(* Logix 5000 AddOnInstructionDefinition export Banner_EZAK2_Param_v4; software revision 33.00; part 2 of 3 *)
(* tags used below, declared in another part *)
   EZAK2 : Banner_EZAK2_v4;
   Port_Data : Banner_IOL_Port_v4;
   Port : DINT;
   Local_Control : DINT;
   Command_Being_Processed : BOOL;
   Update_Archive : BOOL;
   Index_Write_Control : DINT;
   Index_Write_Inprocess : INT;
   Inprocess_Index : DINT;
(* Banner_EZAK2_Param_v4, continued *)

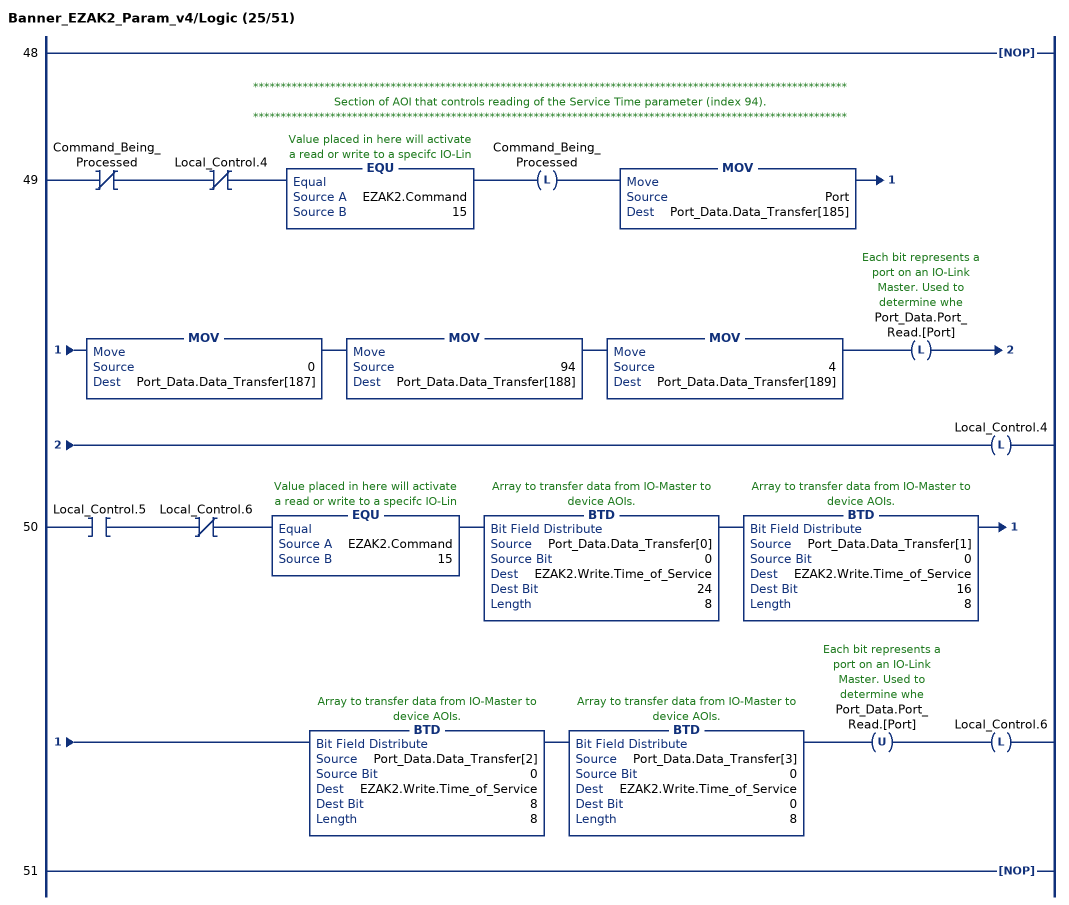
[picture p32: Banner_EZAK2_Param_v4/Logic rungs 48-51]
   48: NOP();
   // ************************************************************************************************************
   // Section of AOI that controls reading of the Service Time parameter (index 94).
   // ************************************************************************************************************
   49: XIO(Command_Being_Processed)XIO(Local_Control.4)EQU(EZAK2.Command,15)OTL(Command_Being_Processed)MOV(Port,Port_Data.Data_Transfer[185])MOV(0,Port_Data.Data_Transfer[187])MOV(94,Port_Data.Data_Transfer[188])MOV(4,Port_Data.Data_Transfer[189])OTL(Port_Data.Port_Read.[Port])OTL(Local_Control.4);
   50: XIC(Local_Control.5)XIO(Local_Control.6)EQU(EZAK2.Command,15)BTD(Port_Data.Data_Transfer[0],0,EZAK2.Write.Time_of_Service,24,8)BTD(Port_Data.Data_Transfer[1],0,EZAK2.Write.Time_of_Service,16,8)BTD(Port_Data.Data_Transfer[2],0,EZAK2.Write.Time_of_Service,8,8)BTD(Port_Data.Data_Transfer[3],0,EZAK2.Write.Time_of_Service,0,8)OTU(Port_Data.Port_Read.[Port])OTL(Local_Control.6);
   51: NOP();
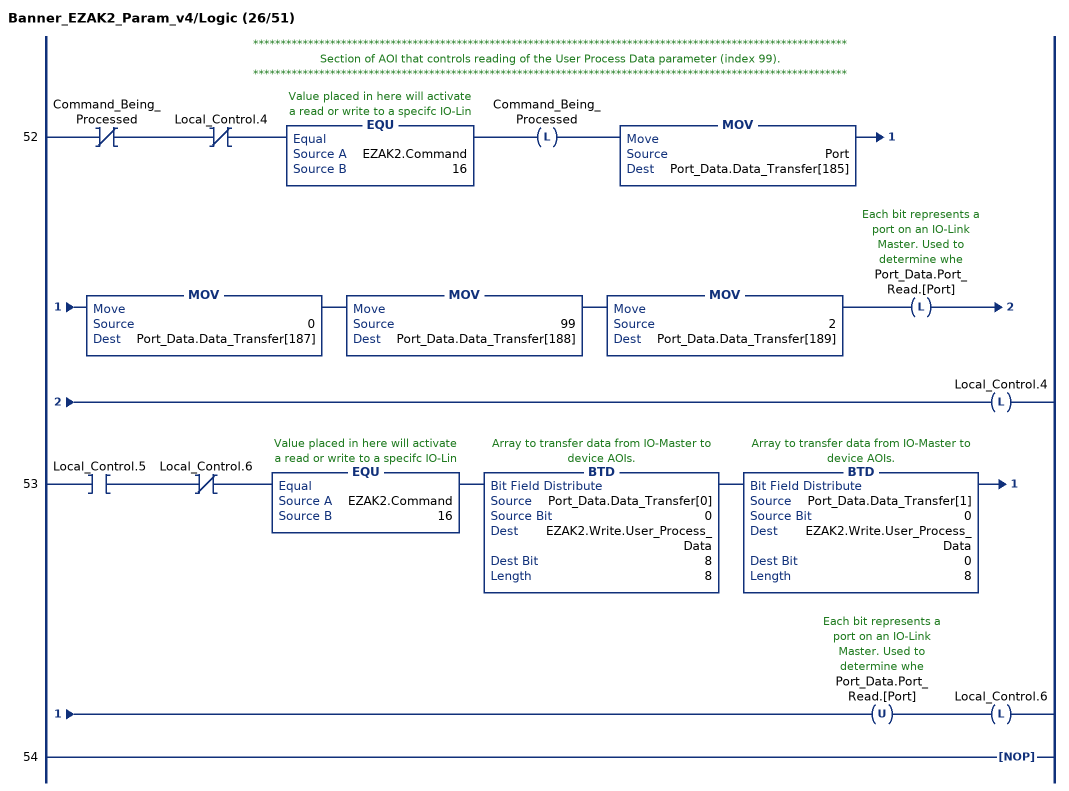
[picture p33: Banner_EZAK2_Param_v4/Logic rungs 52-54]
   // ************************************************************************************************************
   // Section of AOI that controls reading of the User Process Data parameter (index 99).
   // ************************************************************************************************************
   52: XIO(Command_Being_Processed)XIO(Local_Control.4)EQU(EZAK2.Command,16)OTL(Command_Being_Processed)MOV(Port,Port_Data.Data_Transfer[185])MOV(0,Port_Data.Data_Transfer[187])MOV(99,Port_Data.Data_Transfer[188])MOV(2,Port_Data.Data_Transfer[189])OTL(Port_Data.Port_Read.[Port])OTL(Local_Control.4);
   53: XIC(Local_Control.5)XIO(Local_Control.6)EQU(EZAK2.Command,16)BTD(Port_Data.Data_Transfer[0],0,EZAK2.Write.User_Process_Data,8,8)BTD(Port_Data.Data_Transfer[1],0,EZAK2.Write.User_Process_Data,0,8)OTU(Port_Data.Port_Read.[Port])OTL(Local_Control.6);
   54: NOP();
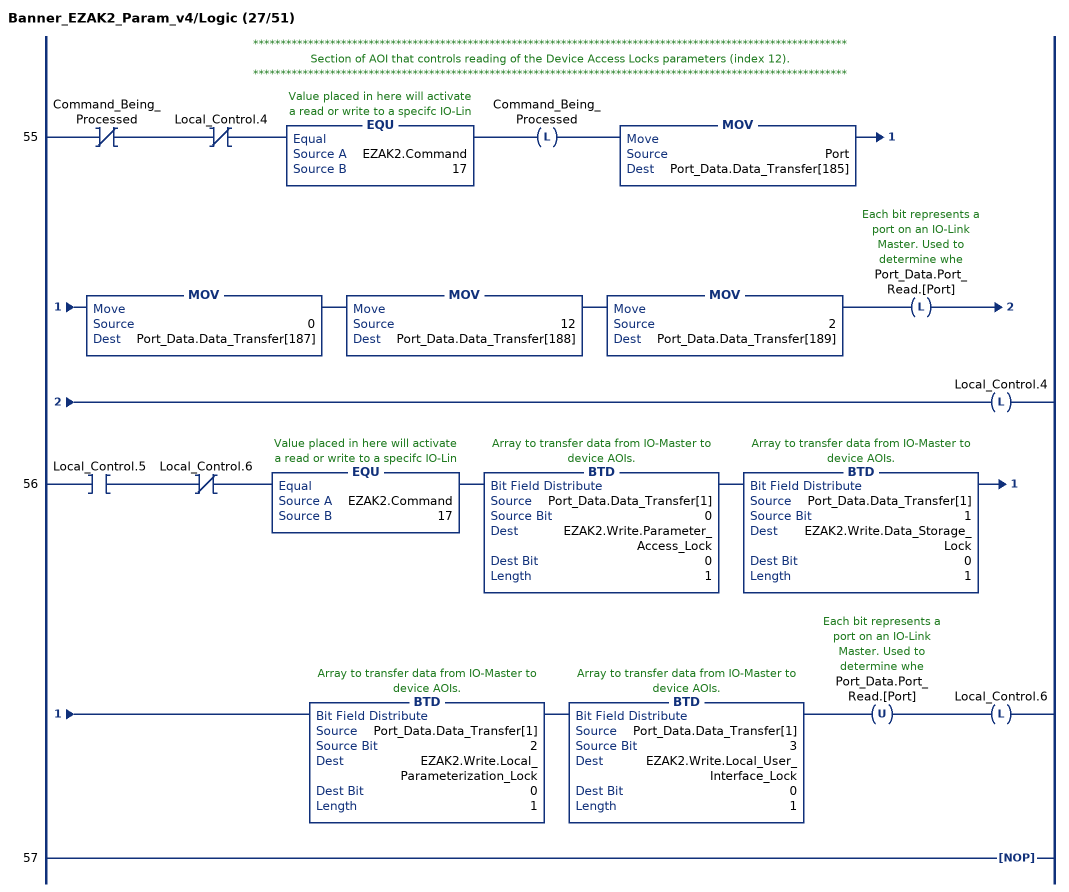
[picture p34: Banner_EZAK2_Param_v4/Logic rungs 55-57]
   // ************************************************************************************************************
   // Section of AOI that controls reading of the Device Access Locks parameters (index 12).
   // ************************************************************************************************************
   55: XIO(Command_Being_Processed)XIO(Local_Control.4)EQU(EZAK2.Command,17)OTL(Command_Being_Processed)MOV(Port,Port_Data.Data_Transfer[185])MOV(0,Port_Data.Data_Transfer[187])MOV(12,Port_Data.Data_Transfer[188])MOV(2,Port_Data.Data_Transfer[189])OTL(Port_Data.Port_Read.[Port])OTL(Local_Control.4);
   56: XIC(Local_Control.5)XIO(Local_Control.6)EQU(EZAK2.Command,17)BTD(Port_Data.Data_Transfer[1],0,EZAK2.Write.Parameter_Access_Lock,0,1)BTD(Port_Data.Data_Transfer[1],1,EZAK2.Write.Data_Storage_Lock,0,1)BTD(Port_Data.Data_Transfer[1],2,EZAK2.Write.Local_Parameterization_Lock,0,1)BTD(Port_Data.Data_Transfer[1],3,EZAK2.Write.Local_User_Interface_Lock,0,1)OTU(Port_Data.Port_Read.[Port])OTL(Local_Control.6);
   57: NOP();
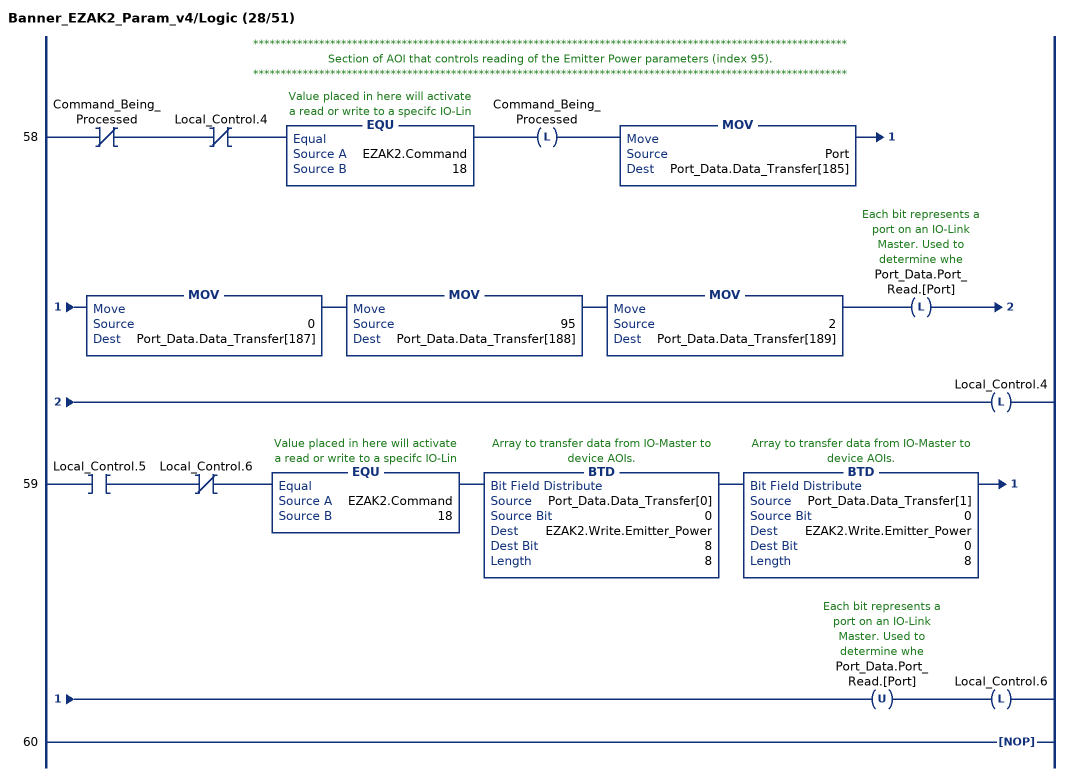
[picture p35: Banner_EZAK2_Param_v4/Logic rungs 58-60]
   // ************************************************************************************************************
   // Section of AOI that controls reading of the Emitter Power parameters (index 95).
   // ************************************************************************************************************
   58: XIO(Command_Being_Processed)XIO(Local_Control.4)EQU(EZAK2.Command,18)OTL(Command_Being_Processed)MOV(Port,Port_Data.Data_Transfer[185])MOV(0,Port_Data.Data_Transfer[187])MOV(95,Port_Data.Data_Transfer[188])MOV(2,Port_Data.Data_Transfer[189])OTL(Port_Data.Port_Read.[Port])OTL(Local_Control.4);
   59: XIC(Local_Control.5)XIO(Local_Control.6)EQU(EZAK2.Command,18)BTD(Port_Data.Data_Transfer[0],0,EZAK2.Write.Emitter_Power,8,8)BTD(Port_Data.Data_Transfer[1],0,EZAK2.Write.Emitter_Power,0,8)OTU(Port_Data.Port_Read.[Port])OTL(Local_Control.6);
   60: NOP();
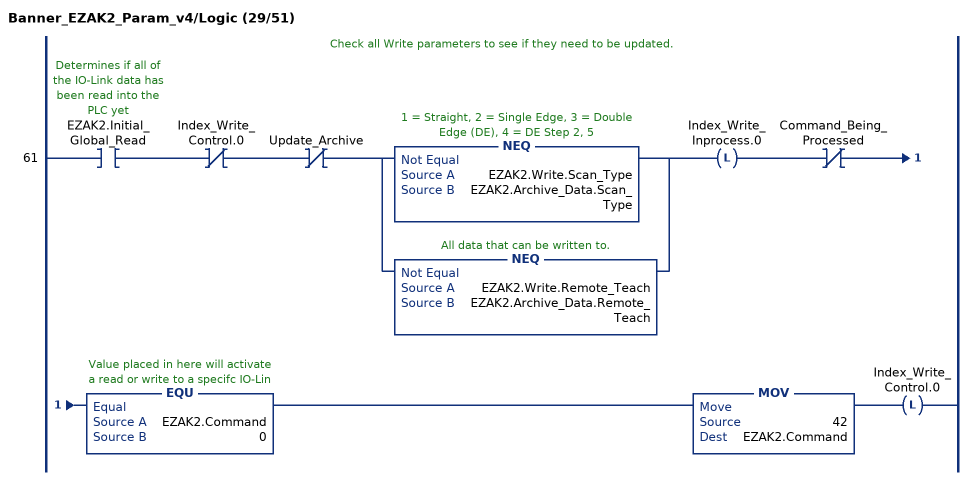
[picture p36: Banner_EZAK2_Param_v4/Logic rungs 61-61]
   // Check all Write parameters to see if they need to be updated.
   61: XIC(EZAK2.Initial_Global_Read)XIO(Index_Write_Control.0)XIO(Update_Archive)[NEQ(EZAK2.Write.Scan_Type,EZAK2.Archive_Data.Scan_Type) ,NEQ(EZAK2.Write.Remote_Teach,EZAK2.Archive_Data.Remote_Teach) ]OTL(Index_Write_Inprocess.0)XIO(Command_Being_Processed)EQU(EZAK2.Command,0)MOV(42,EZAK2.Command)OTL(Index_Write_Control.0);
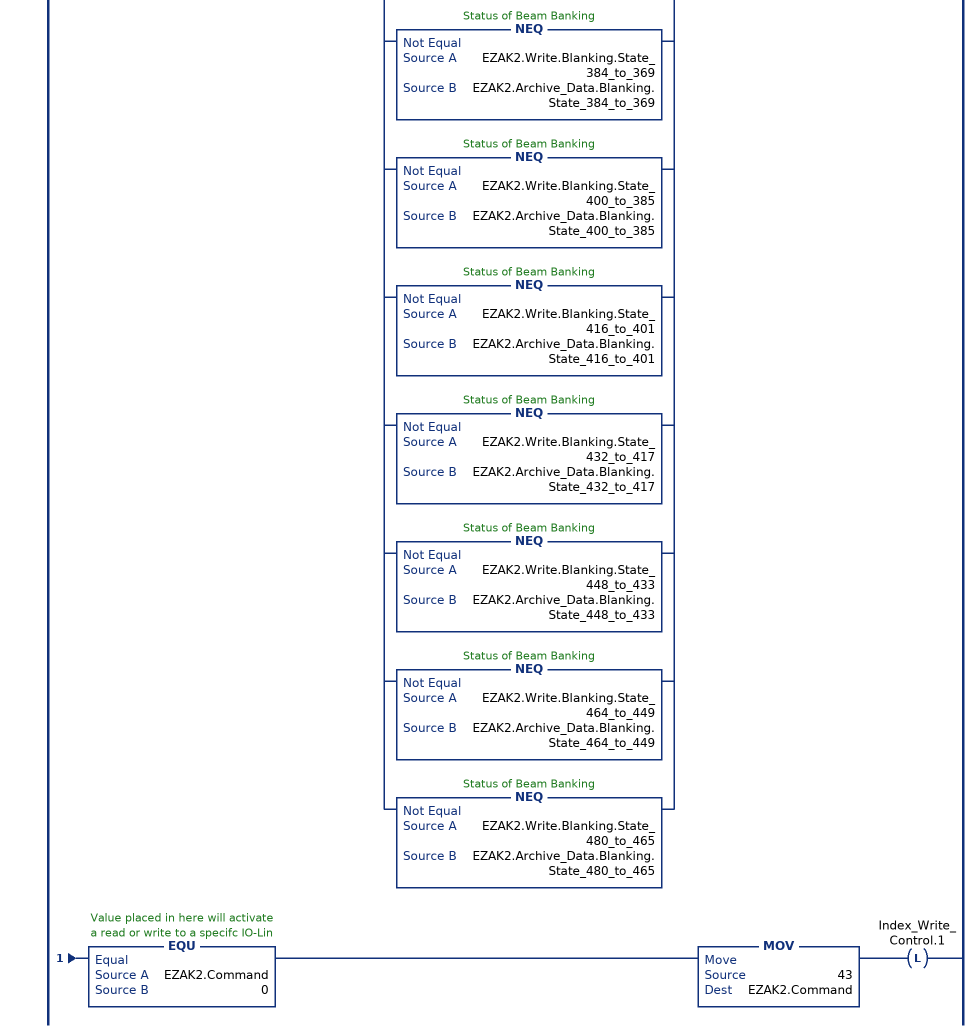
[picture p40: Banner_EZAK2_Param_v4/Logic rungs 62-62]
   62: XIC(EZAK2.Initial_Global_Read)XIO(Index_Write_Control.1)XIO(Update_Archive)[NEQ(EZAK2.Write.Blanking.State_16_to_1,EZAK2.Archive_Data.Blanking.State_16_to_1) ,NEQ(EZAK2.Write.Blanking.State_32_to_17,EZAK2.Archive_Data.Blanking.State_32_to_17) ,NEQ(EZAK2.Write.Blanking.State_48_to_33,EZAK2.Archive_Data.Blanking.State_48_to_33) ,NEQ(EZAK2.Write.Blanking.State_64_to_49,EZAK2.Archive_Data.Blanking.State_64_to_49) ,NEQ(EZAK2.Write.Blanking.State_80_to_65,EZAK2.Archive_Data.Blanking.State_80_to_65) ,NEQ(EZAK2.Write.Blanking.State_96_to_81,EZAK2.Archive_Data.Blanking.State_96_to_81) ,NEQ(EZAK2.Write.Blanking.State_112_to_97,EZAK2.Archive_Data.Blanking.State_112_to_97) ,NEQ(EZAK2.Write.Blanking.State_128_to_113,EZAK2.Archive_Data.Blanking.State_128_to_113) ,NEQ(EZAK2.Write.Blanking.State_144_to_129,EZAK2.Archive_Data.Blanking.State_144_to_129) ,NEQ(EZAK2.Write.Blanking.State_160_to_145,EZAK2.Archive_Data.Blanking.State_160_to_145) ,NEQ(EZAK2.Write.Blanking.State_176_to_161,EZAK2.Archive_Data.Blanking.State_176_to_161) ,NEQ(EZAK2.Write.Blanking.State_192_to_177,EZAK2.Archive_Data.Blanking.State_192_to_177) ,NEQ(EZAK2.Write.Blanking.State_208_to_193,EZAK2.Archive_Data.Blanking.State_208_to_193) ,NEQ(EZAK2.Write.Blanking.State_224_to_209,EZAK2.Archive_Data.Blanking.State_224_to_209) ,NEQ(EZAK2.Write.Blanking.State_240_to_225,EZAK2.Archive_Data.Blanking.State_240_to_225) ,NEQ(EZAK2.Write.Blanking.State_256_to_241,EZAK2.Archive_Data.Blanking.State_256_to_241) ,NEQ(EZAK2.Write.Blanking.State_272_to_257,EZAK2.Archive_Data.Blanking.State_272_to_257) ,NEQ(EZAK2.Write.Blanking.State_288_to_273,EZAK2.Archive_Data.Blanking.State_288_to_273) ,NEQ(EZAK2.Write.Blanking.State_304_to_289,EZAK2.Archive_Data.Blanking.State_304_to_289) ,NEQ(EZAK2.Write.Blanking.State_320_to_305,EZAK2.Archive_Data.Blanking.State_320_to_305) ,NEQ(EZAK2.Write.Blanking.State_336_to_321,EZAK2.Archive_Data.Blanking.State_336_to_321) ,NEQ(EZAK2.Write.Blanking.State_352_to_337,EZAK2.Archive_Data.Blanking.State_352_to_337) ,NEQ(EZAK2.Write.Blanking.State_368_to_353,EZAK2.Archive_Data.Blanking.State_368_to_353) ,NEQ(EZAK2.Write.Blanking.State_384_to_369,EZAK2.Archive_Data.Blanking.State_384_to_369) ,NEQ(EZAK2.Write.Blanking.State_400_to_385,EZAK2.Archive_Data.Blanking.State_400_to_385) ,NEQ(EZAK2.Write.Blanking.State_416_to_401,EZAK2.Archive_Data.Blanking.State_416_to_401) ,NEQ(EZAK2.Write.Blanking.State_432_to_417,EZAK2.Archive_Data.Blanking.State_432_to_417) ,NEQ(EZAK2.Write.Blanking.State_448_to_433,EZAK2.Archive_Data.Blanking.State_448_to_433) ,NEQ(EZAK2.Write.Blanking.State_464_to_449,EZAK2.Archive_Data.Blanking.State_464_to_449) ,NEQ(EZAK2.Write.Blanking.State_480_to_465,EZAK2.Archive_Data.Blanking.State_480_to_465) ]OTL(Index_Write_Inprocess.1)XIO(Command_Being_Processed)EQU(EZAK2.Command,0)MOV(43,EZAK2.Command)OTL(Index_Write_Control.1);
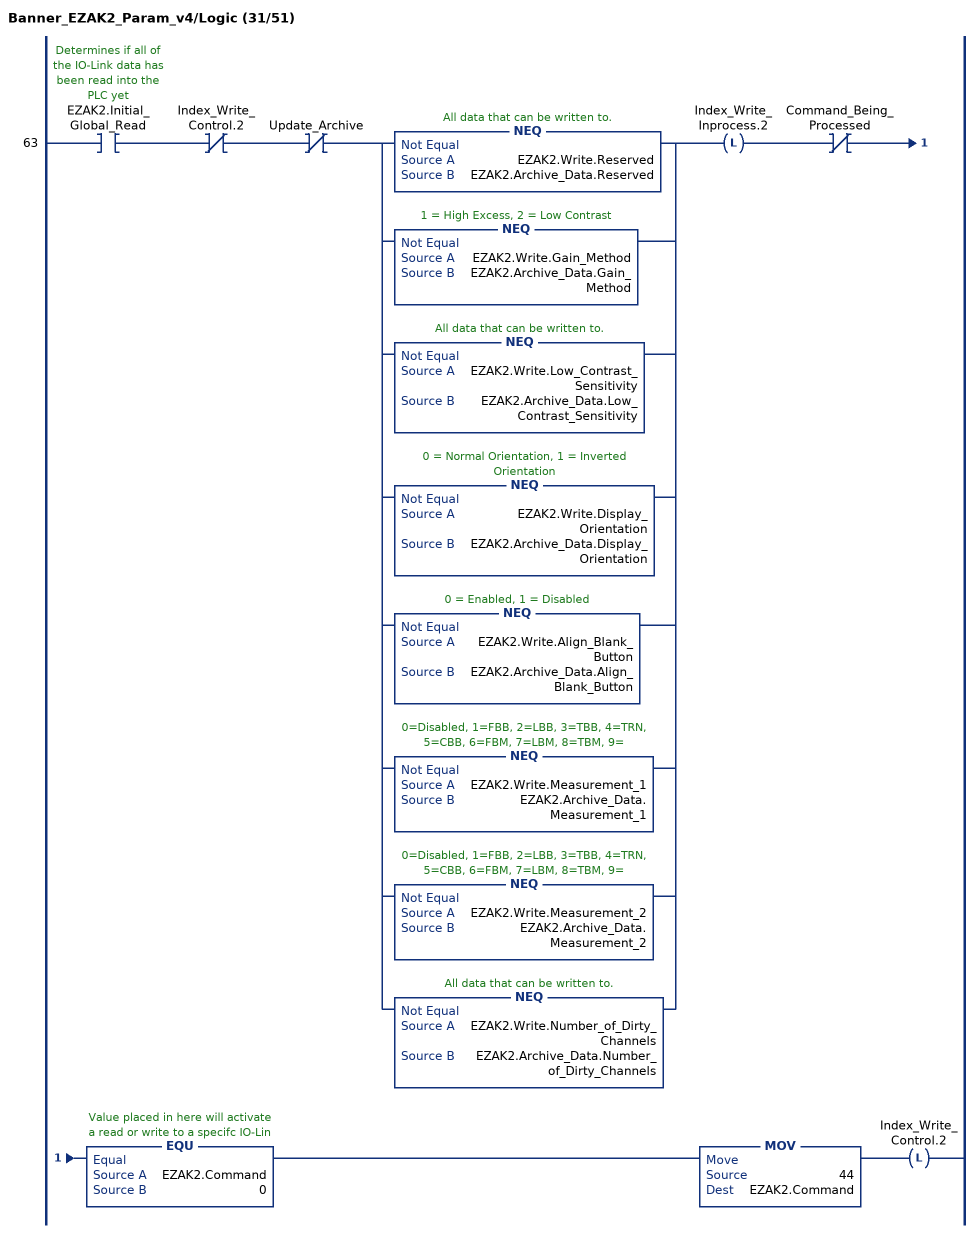
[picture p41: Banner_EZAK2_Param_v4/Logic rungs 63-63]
   63: XIC(EZAK2.Initial_Global_Read)XIO(Index_Write_Control.2)XIO(Update_Archive)[NEQ(EZAK2.Write.Reserved,EZAK2.Archive_Data.Reserved) ,NEQ(EZAK2.Write.Gain_Method,EZAK2.Archive_Data.Gain_Method) ,NEQ(EZAK2.Write.Low_Contrast_Sensitivity,EZAK2.Archive_Data.Low_Contrast_Sensitivity) ,NEQ(EZAK2.Write.Display_Orientation,EZAK2.Archive_Data.Display_Orientation) ,NEQ(EZAK2.Write.Align_Blank_Button,EZAK2.Archive_Data.Align_Blank_Button) ,NEQ(EZAK2.Write.Measurement_1,EZAK2.Archive_Data.Measurement_1) ,NEQ(EZAK2.Write.Measurement_2,EZAK2.Archive_Data.Measurement_2) ,NEQ(EZAK2.Write.Number_of_Dirty_Channels,EZAK2.Archive_Data.Number_of_Dirty_Channels) ]OTL(Index_Write_Inprocess.2)XIO(Command_Being_Processed)EQU(EZAK2.Command,0)MOV(44,EZAK2.Command)OTL(Index_Write_Control.2);
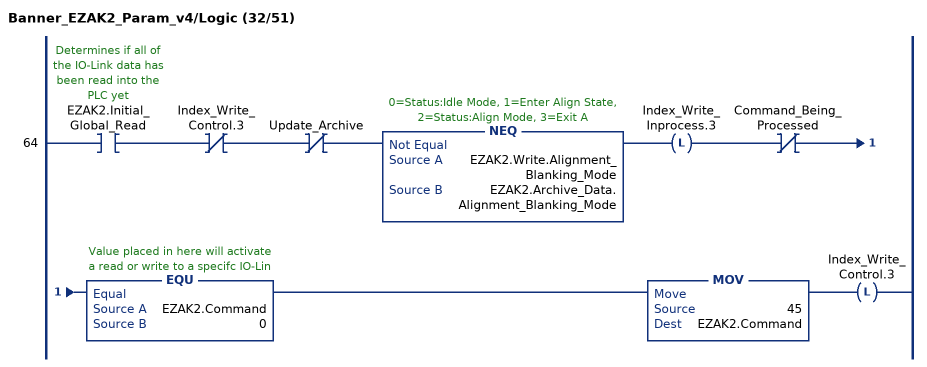
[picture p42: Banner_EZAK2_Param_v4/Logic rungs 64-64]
   64: XIC(EZAK2.Initial_Global_Read)XIO(Index_Write_Control.3)XIO(Update_Archive)NEQ(EZAK2.Write.Alignment_Blanking_Mode,EZAK2.Archive_Data.Alignment_Blanking_Mode)OTL(Index_Write_Inprocess.3)XIO(Command_Being_Processed)EQU(EZAK2.Command,0)MOV(45,EZAK2.Command)OTL(Index_Write_Control.3);
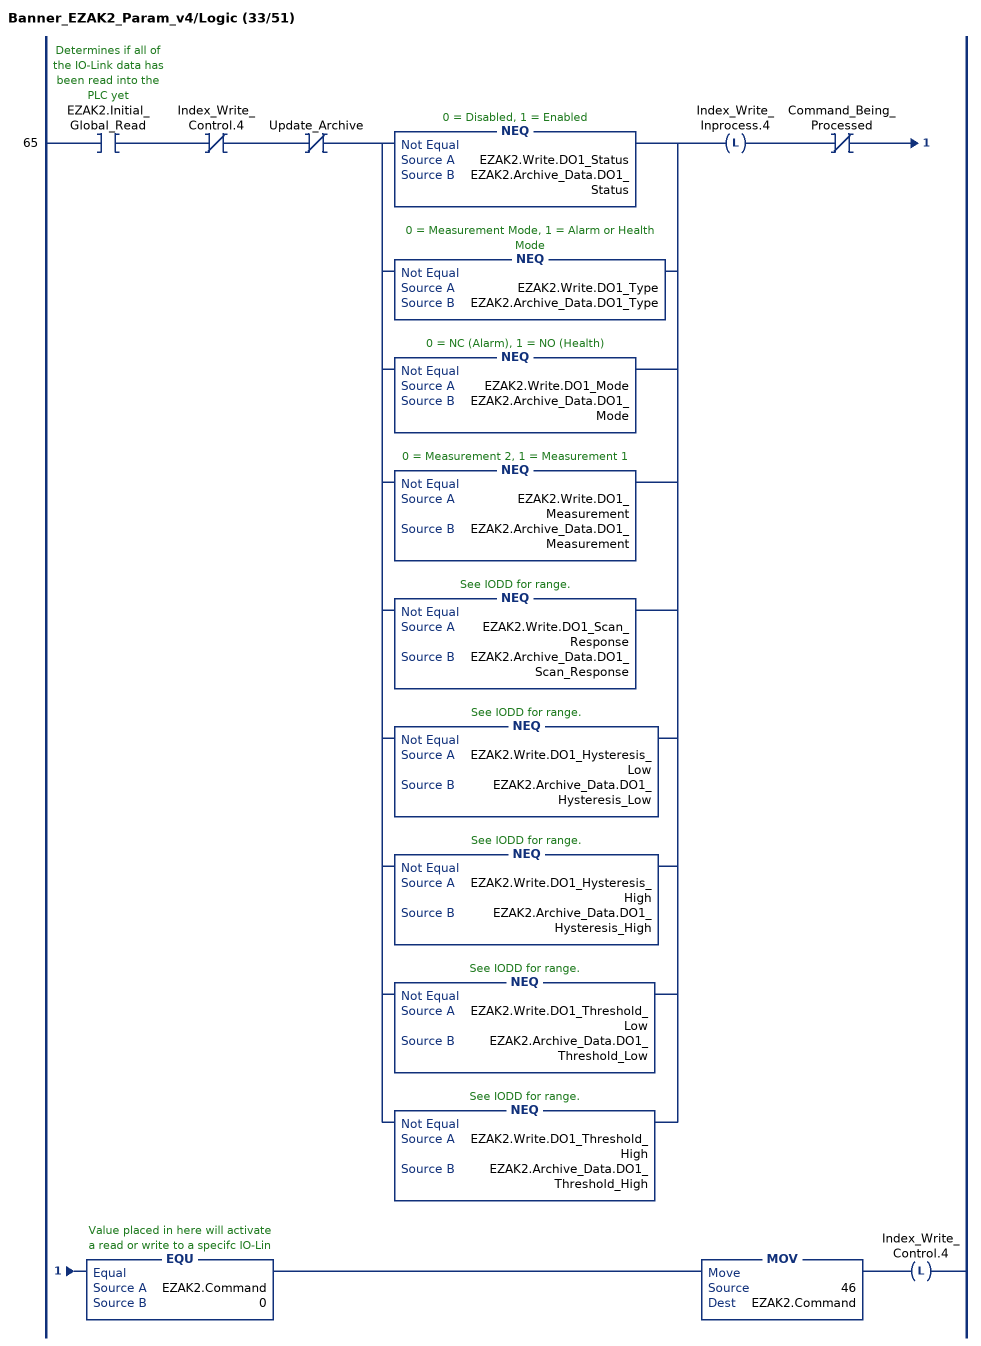
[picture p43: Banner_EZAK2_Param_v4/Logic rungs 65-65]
   65: XIC(EZAK2.Initial_Global_Read)XIO(Index_Write_Control.4)XIO(Update_Archive)[NEQ(EZAK2.Write.DO1_Status,EZAK2.Archive_Data.DO1_Status) ,NEQ(EZAK2.Write.DO1_Type,EZAK2.Archive_Data.DO1_Type) ,NEQ(EZAK2.Write.DO1_Mode,EZAK2.Archive_Data.DO1_Mode) ,NEQ(EZAK2.Write.DO1_Measurement,EZAK2.Archive_Data.DO1_Measurement) ,NEQ(EZAK2.Write.DO1_Scan_Response,EZAK2.Archive_Data.DO1_Scan_Response) ,NEQ(EZAK2.Write.DO1_Hysteresis_Low,EZAK2.Archive_Data.DO1_Hysteresis_Low) ,NEQ(EZAK2.Write.DO1_Hysteresis_High,EZAK2.Archive_Data.DO1_Hysteresis_High) ,NEQ(EZAK2.Write.DO1_Threshold_Low,EZAK2.Archive_Data.DO1_Threshold_Low) ,NEQ(EZAK2.Write.DO1_Threshold_High,EZAK2.Archive_Data.DO1_Threshold_High) ]OTL(Index_Write_Inprocess.4)XIO(Command_Being_Processed)EQU(EZAK2.Command,0)MOV(46,EZAK2.Command)OTL(Index_Write_Control.4);
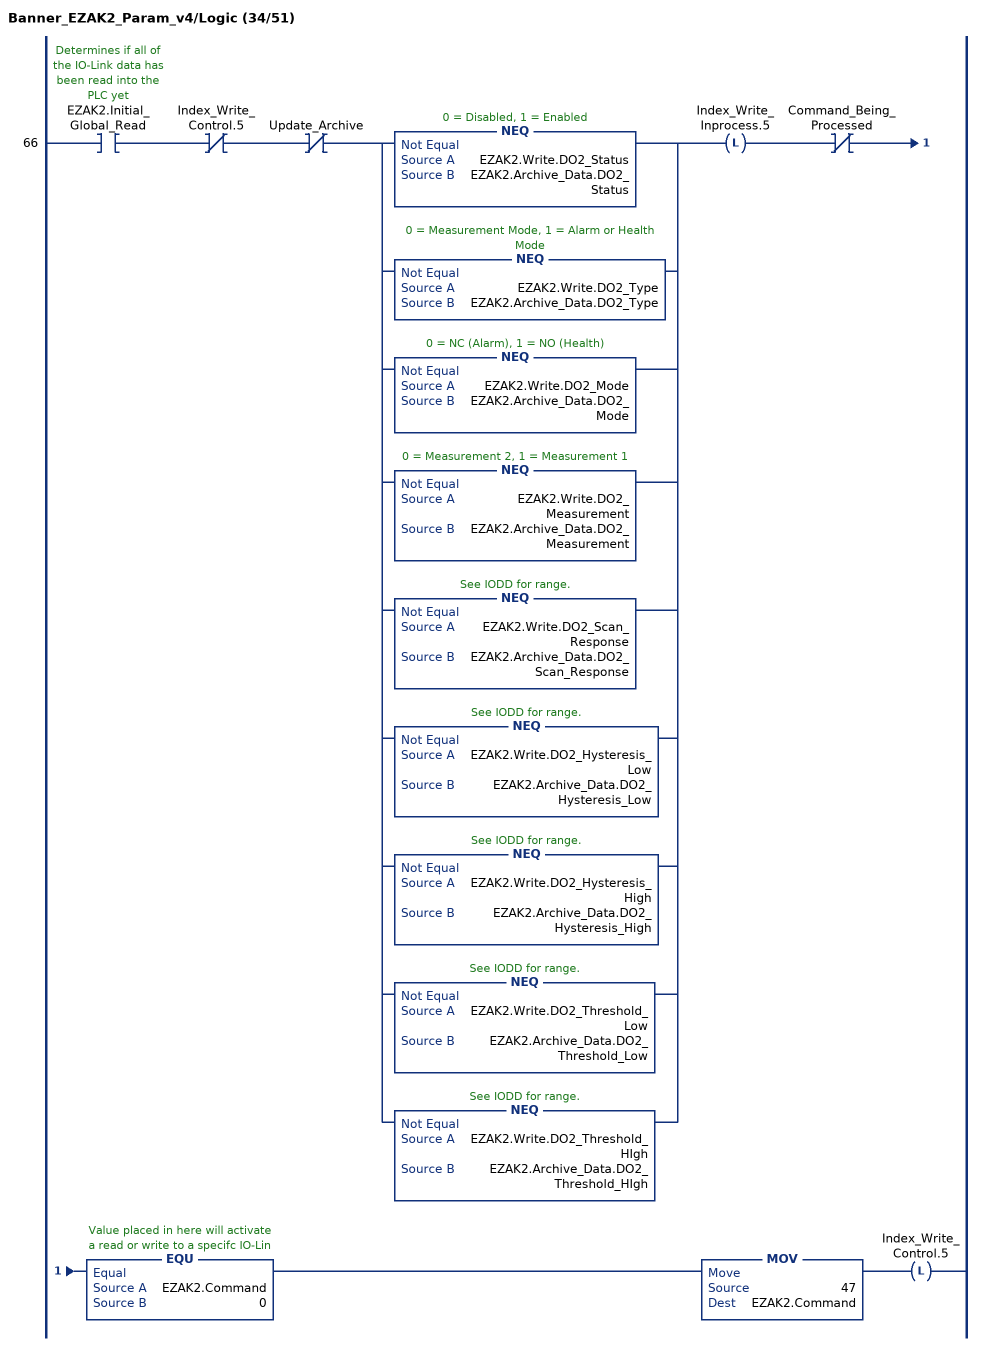
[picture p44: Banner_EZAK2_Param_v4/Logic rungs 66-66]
   66: XIC(EZAK2.Initial_Global_Read)XIO(Index_Write_Control.5)XIO(Update_Archive)[NEQ(EZAK2.Write.DO2_Status,EZAK2.Archive_Data.DO2_Status) ,NEQ(EZAK2.Write.DO2_Type,EZAK2.Archive_Data.DO2_Type) ,NEQ(EZAK2.Write.DO2_Mode,EZAK2.Archive_Data.DO2_Mode) ,NEQ(EZAK2.Write.DO2_Measurement,EZAK2.Archive_Data.DO2_Measurement) ,NEQ(EZAK2.Write.DO2_Scan_Response,EZAK2.Archive_Data.DO2_Scan_Response) ,NEQ(EZAK2.Write.DO2_Hysteresis_Low,EZAK2.Archive_Data.DO2_Hysteresis_Low) ,NEQ(EZAK2.Write.DO2_Hysteresis_High,EZAK2.Archive_Data.DO2_Hysteresis_High) ,NEQ(EZAK2.Write.DO2_Threshold_Low,EZAK2.Archive_Data.DO2_Threshold_Low) ,NEQ(EZAK2.Write.DO2_Threshold_HIgh,EZAK2.Archive_Data.DO2_Threshold_HIgh) ]OTL(Index_Write_Inprocess.5)XIO(Command_Being_Processed)EQU(EZAK2.Command,0)MOV(47,EZAK2.Command)OTL(Index_Write_Control.5);
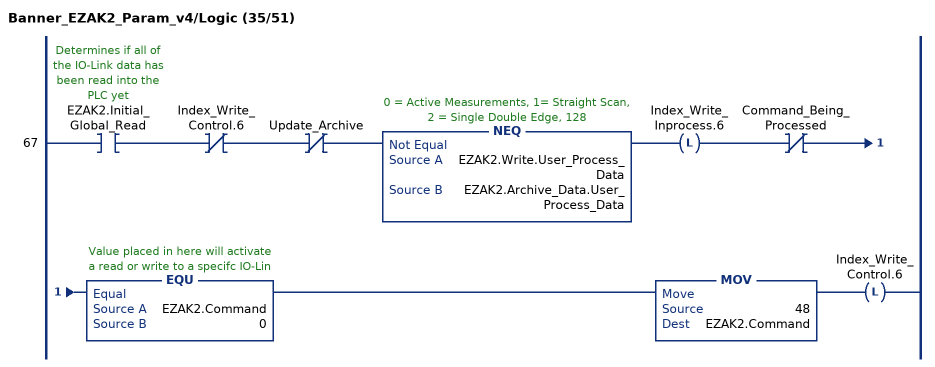
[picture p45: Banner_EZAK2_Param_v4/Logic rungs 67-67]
   67: XIC(EZAK2.Initial_Global_Read)XIO(Index_Write_Control.6)XIO(Update_Archive)NEQ(EZAK2.Write.User_Process_Data,EZAK2.Archive_Data.User_Process_Data)OTL(Index_Write_Inprocess.6)XIO(Command_Being_Processed)EQU(EZAK2.Command,0)MOV(48,EZAK2.Command)OTL(Index_Write_Control.6);
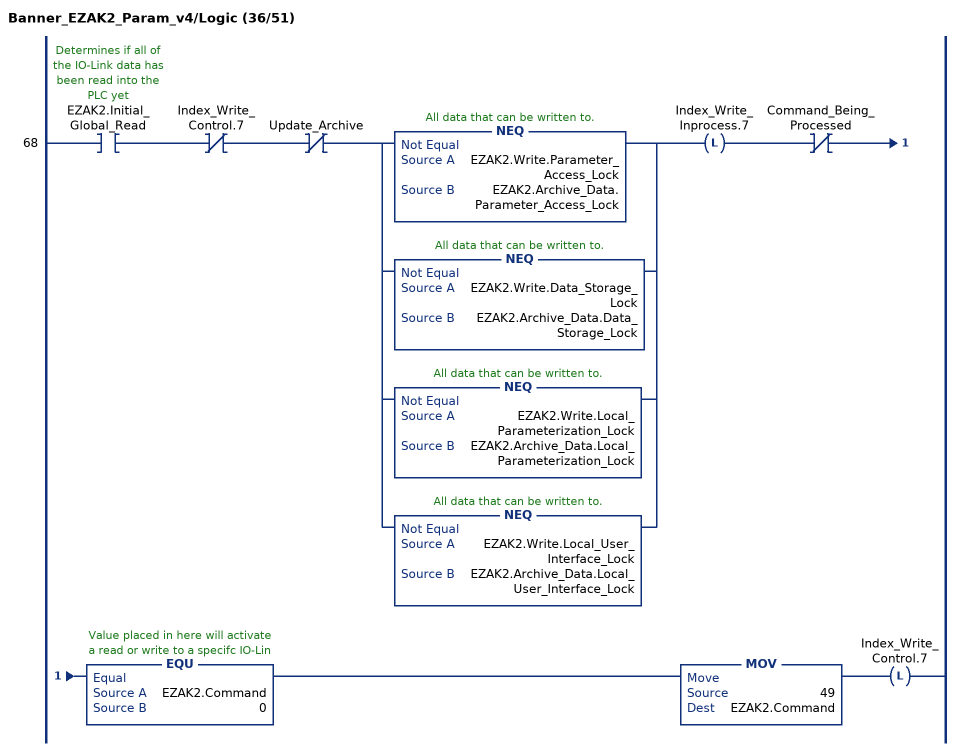
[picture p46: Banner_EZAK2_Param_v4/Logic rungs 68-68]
   68: XIC(EZAK2.Initial_Global_Read)XIO(Index_Write_Control.7)XIO(Update_Archive)[NEQ(EZAK2.Write.Parameter_Access_Lock,EZAK2.Archive_Data.Parameter_Access_Lock) ,NEQ(EZAK2.Write.Data_Storage_Lock,EZAK2.Archive_Data.Data_Storage_Lock) ,NEQ(EZAK2.Write.Local_Parameterization_Lock,EZAK2.Archive_Data.Local_Parameterization_Lock) ,NEQ(EZAK2.Write.Local_User_Interface_Lock,EZAK2.Archive_Data.Local_User_Interface_Lock) ]OTL(Index_Write_Inprocess.7)XIO(Command_Being_Processed)EQU(EZAK2.Command,0)MOV(49,EZAK2.Command)OTL(Index_Write_Control.7);
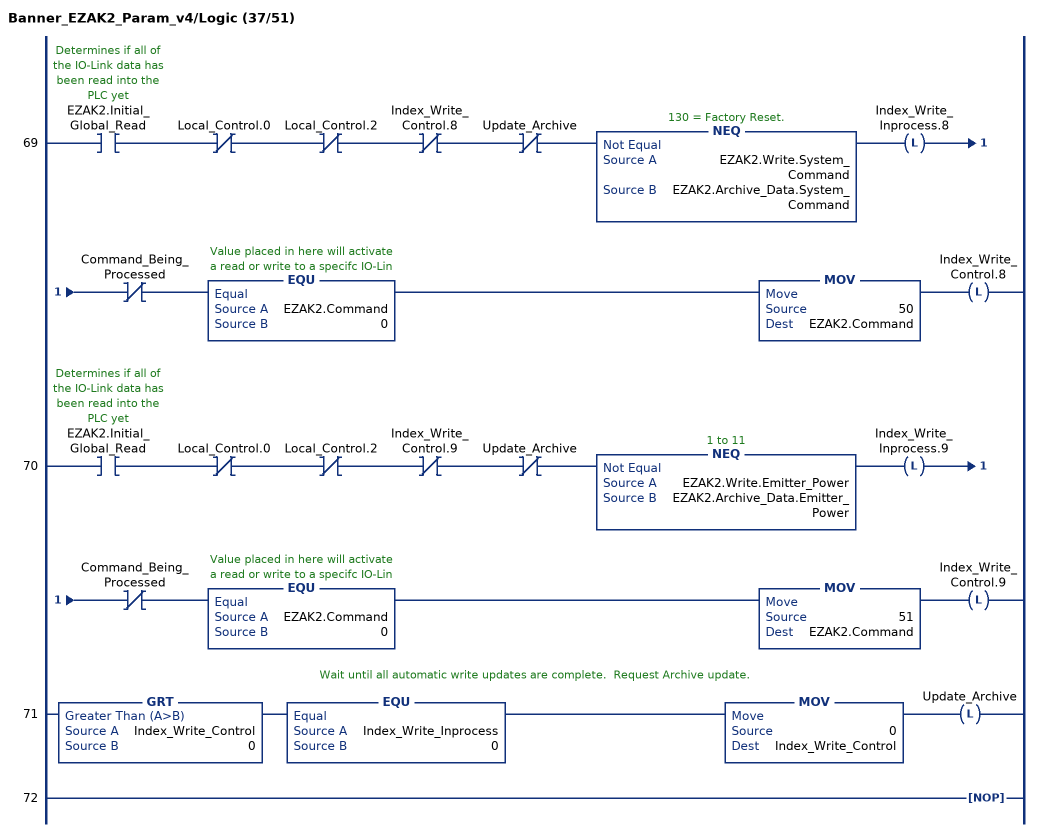
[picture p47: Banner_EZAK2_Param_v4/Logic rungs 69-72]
   69: XIC(EZAK2.Initial_Global_Read)XIO(Local_Control.0)XIO(Local_Control.2)XIO(Index_Write_Control.8)XIO(Update_Archive)NEQ(EZAK2.Write.System_Command,EZAK2.Archive_Data.System_Command)OTL(Index_Write_Inprocess.8)XIO(Command_Being_Processed)EQU(EZAK2.Command,0)MOV(50,EZAK2.Command)OTL(Index_Write_Control.8);
   70: XIC(EZAK2.Initial_Global_Read)XIO(Local_Control.0)XIO(Local_Control.2)XIO(Index_Write_Control.9)XIO(Update_Archive)NEQ(EZAK2.Write.Emitter_Power,EZAK2.Archive_Data.Emitter_Power)OTL(Index_Write_Inprocess.9)XIO(Command_Being_Processed)EQU(EZAK2.Command,0)MOV(51,EZAK2.Command)OTL(Index_Write_Control.9);
   // Wait until all automatic write updates are complete.  Request Archive update.
   71: GRT(Index_Write_Control,0)EQU(Index_Write_Inprocess,0)MOV(0,Index_Write_Control)OTL(Update_Archive);
   72: NOP();
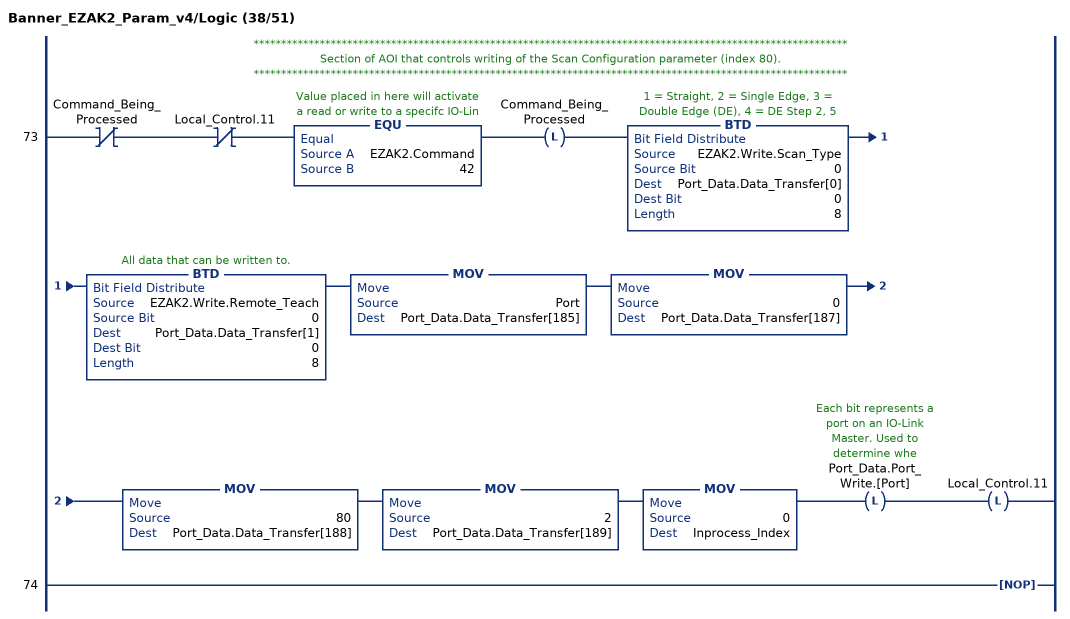
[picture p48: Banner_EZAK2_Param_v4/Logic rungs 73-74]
   // ************************************************************************************************************
   // Section of AOI that controls writing of the Scan Configuration parameter (index 80).
   // ************************************************************************************************************
   73: XIO(Command_Being_Processed)XIO(Local_Control.11)EQU(EZAK2.Command,42)OTL(Command_Being_Processed)BTD(EZAK2.Write.Scan_Type,0,Port_Data.Data_Transfer[0],0,8)BTD(EZAK2.Write.Remote_Teach,0,Port_Data.Data_Transfer[1],0,8)MOV(Port,Port_Data.Data_Transfer[185])MOV(0,Port_Data.Data_Transfer[187])MOV(80,Port_Data.Data_Transfer[188])MOV(2,Port_Data.Data_Transfer[189])MOV(0,Inprocess_Index)OTL(Port_Data.Port_Write.[Port])OTL(Local_Control.11);
   74: NOP();
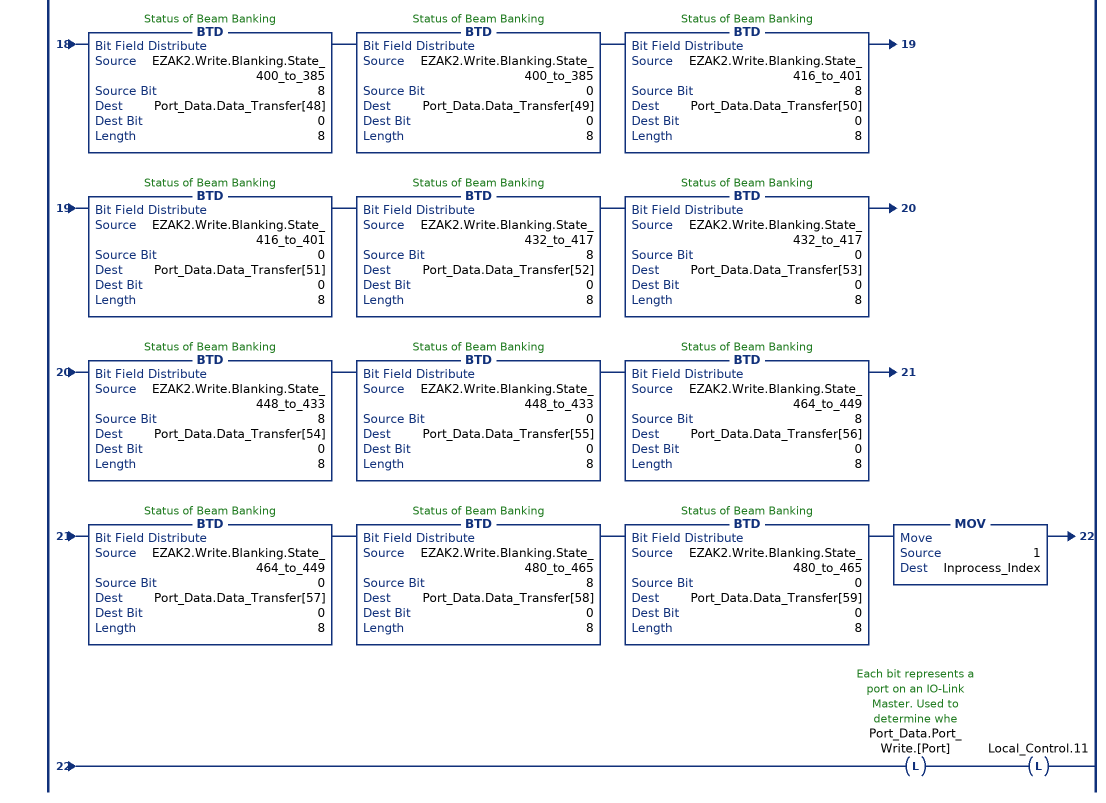
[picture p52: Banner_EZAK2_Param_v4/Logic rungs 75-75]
   // ************************************************************************************************************
   // Section of AOI that controls writing of the Blanking Configuration parameter (index 81).
   // ************************************************************************************************************
   75: XIO(Command_Being_Processed)XIO(Local_Control.11)EQU(EZAK2.Command,43)OTL(Command_Being_Processed)MOV(Port,Port_Data.Data_Transfer[185])MOV(0,Port_Data.Data_Transfer[187])MOV(81,Port_Data.Data_Transfer[188])MOV(60,Port_Data.Data_Transfer[189])BTD(EZAK2.Write.Blanking.State_16_to_1,8,Port_Data.Data_Transfer[0],0,8)BTD(EZAK2.Write.Blanking.State_16_to_1,0,Port_Data.Data_Transfer[1],0,8)BTD(EZAK2.Write.Blanking.State_32_to_17,8,Port_Data.Data_Transfer[2],0,8)BTD(EZAK2.Write.Blanking.State_32_to_17,0,Port_Data.Data_Transfer[3],0,8)BTD(EZAK2.Write.Blanking.State_48_to_33,8,Port_Data.Data_Transfer[4],0,8)BTD(EZAK2.Write.Blanking.State_48_to_33,0,Port_Data.Data_Transfer[5],0,8)BTD(EZAK2.Write.Blanking.State_64_to_49,8,Port_Data.Data_Transfer[6],0,8)BTD(EZAK2.Write.Blanking.State_64_to_49,0,Port_Data.Data_Transfer[7],0,8)BTD(EZAK2.Write.Blanking.State_80_to_65,8,Port_Data.Data_Transfer[8],0,8)BTD(EZAK2.Write.Blanking.State_80_to_65,0,Port_Data.Data_Transfer[9],0,8)BTD(EZAK2.Write.Blanking.State_96_to_81,8,Port_Data.Data_Transfer[10],0,8)BTD(EZAK2.Write.Blanking.State_96_to_81,0,Port_Data.Data_Transfer[11],0,8)BTD(EZAK2.Write.Blanking.State_112_to_97,8,Port_Data.Data_Transfer[12],0,8)BTD(EZAK2.Write.Blanking.State_112_to_97,0,Port_Data.Data_Transfer[13],0,8)BTD(EZAK2.Write.Blanking.State_128_to_113,8,Port_Data.Data_Transfer[14],0,8)BTD(EZAK2.Write.Blanking.State_128_to_113,0,Port_Data.Data_Transfer[15],0,8)BTD(EZAK2.Write.Blanking.State_144_to_129,8,Port_Data.Data_Transfer[16],0,8)BTD(EZAK2.Write.Blanking.State_144_to_129,0,Port_Data.Data_Transfer[17],0,8)BTD(EZAK2.Write.Blanking.State_160_to_145,8,Port_Data.Data_Transfer[18],0,8)BTD(EZAK2.Write.Blanking.State_160_to_145,0,Port_Data.Data_Transfer[19],0,8)BTD(EZAK2.Write.Blanking.State_176_to_161,8,Port_Data.Data_Transfer[20],0,8)BTD(EZAK2.Write.Blanking.State_176_to_161,0,Port_Data.Data_Transfer[21],0,8)BTD(EZAK2.Write.Blanking.State_192_to_177,8,Port_Data.Data_Transfer[22],0,8)BTD(EZAK2.Write.Blanking.State_192_to_177,0,Port_Data.Data_Transfer[23],0,8)BTD(EZAK2.Write.Blanking.State_208_to_193,8,Port_Data.Data_Transfer[24],0,8)BTD(EZAK2.Write.Blanking.State_208_to_193,0,Port_Data.Data_Transfer[25],0,8)BTD(EZAK2.Write.Blanking.State_224_to_209,8,Port_Data.Data_Transfer[26],0,8)BTD(EZAK2.Write.Blanking.State_224_to_209,0,Port_Data.Data_Transfer[27],0,8)BTD(EZAK2.Write.Blanking.State_240_to_225,8,Port_Data.Data_Transfer[28],0,8)BTD(EZAK2.Write.Blanking.State_240_to_225,0,Port_Data.Data_Transfer[29],0,8)BTD(EZAK2.Write.Blanking.State_256_to_241,8,Port_Data.Data_Transfer[30],0,8)BTD(EZAK2.Write.Blanking.State_256_to_241,0,Port_Data.Data_Transfer[31],0,8)BTD(EZAK2.Write.Blanking.State_272_to_257,8,Port_Data.Data_Transfer[32],0,8)BTD(EZAK2.Write.Blanking.State_272_to_257,0,Port_Data.Data_Transfer[33],0,8)BTD(EZAK2.Write.Blanking.State_288_to_273,8,Port_Data.Data_Transfer[34],0,8)BTD(EZAK2.Write.Blanking.State_288_to_273,0,Port_Data.Data_Transfer[35],0,8)BTD(EZAK2.Write.Blanking.State_304_to_289,8,Port_Data.Data_Transfer[36],0,8)BTD(EZAK2.Write.Blanking.State_304_to_289,0,Port_Data.Data_Transfer[37],0,8)BTD(EZAK2.Write.Blanking.State_320_to_305,8,Port_Data.Data_Transfer[38],0,8)BTD(EZAK2.Write.Blanking.State_320_to_305,0,Port_Data.Data_Transfer[39],0,8)BTD(EZAK2.Write.Blanking.State_336_to_321,8,Port_Data.Data_Transfer[40],0,8)BTD(EZAK2.Write.Blanking.State_336_to_321,0,Port_Data.Data_Transfer[41],0,8)BTD(EZAK2.Write.Blanking.State_352_to_337,8,Port_Data.Data_Transfer[42],0,8)BTD(EZAK2.Write.Blanking.State_352_to_337,0,Port_Data.Data_Transfer[43],0,8)BTD(EZAK2.Write.Blanking.State_368_to_353,8,Port_Data.Data_Transfer[44],0,8)BTD(EZAK2.Write.Blanking.State_368_to_353,0,Port_Data.Data_Transfer[45],0,8)BTD(EZAK2.Write.Blanking.State_384_to_369,8,Port_Data.Data_Transfer[46],0,8)BTD(EZAK2.Write.Blanking.State_384_to_369,0,Port_Data.Data_Transfer[47],0,8)BTD(EZAK2.Write.Blanking.State_400_to_385,8,Port_Data.Data_Transfer[48],0,8)BTD(EZAK2.Write.Blanking.State_400_to_385,0,Port_Data.Data_Transfer[49],0,8)BTD(EZAK2.Write.Blanking.State_416_to_401,8,Port_Data.Data_Transfer[50],0,8)BTD(EZAK2.Write.Blanking.State_416_to_401,0,Port_Data.Data_Transfer[51],0,8)BTD(EZAK2.Write.Blanking.State_432_to_417,8,Port_Data.Data_Transfer[52],0,8)BTD(EZAK2.Write.Blanking.State_432_to_417,0,Port_Data.Data_Transfer[53],0,8)BTD(EZAK2.Write.Blanking.State_448_to_433,8,Port_Data.Data_Transfer[54],0,8)BTD(EZAK2.Write.Blanking.State_448_to_433,0,Port_Data.Data_Transfer[55],0,8)BTD(EZAK2.Write.Blanking.State_464_to_449,8,Port_Data.Data_Transfer[56],0,8)BTD(EZAK2.Write.Blanking.State_464_to_449,0,Port_Data.Data_Transfer[57],0,8)BTD(EZAK2.Write.Blanking.State_480_to_465,8,Port_Data.Data_Transfer[58],0,8)BTD(EZAK2.Write.Blanking.State_480_to_465,0,Port_Data.Data_Transfer[59],0,8)MOV(1,Inprocess_Index)OTL(Port_Data.Port_Write.[Port])OTL(Local_Control.11);
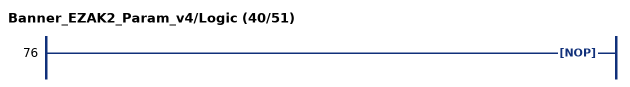
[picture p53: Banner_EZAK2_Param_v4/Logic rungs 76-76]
   76: NOP();
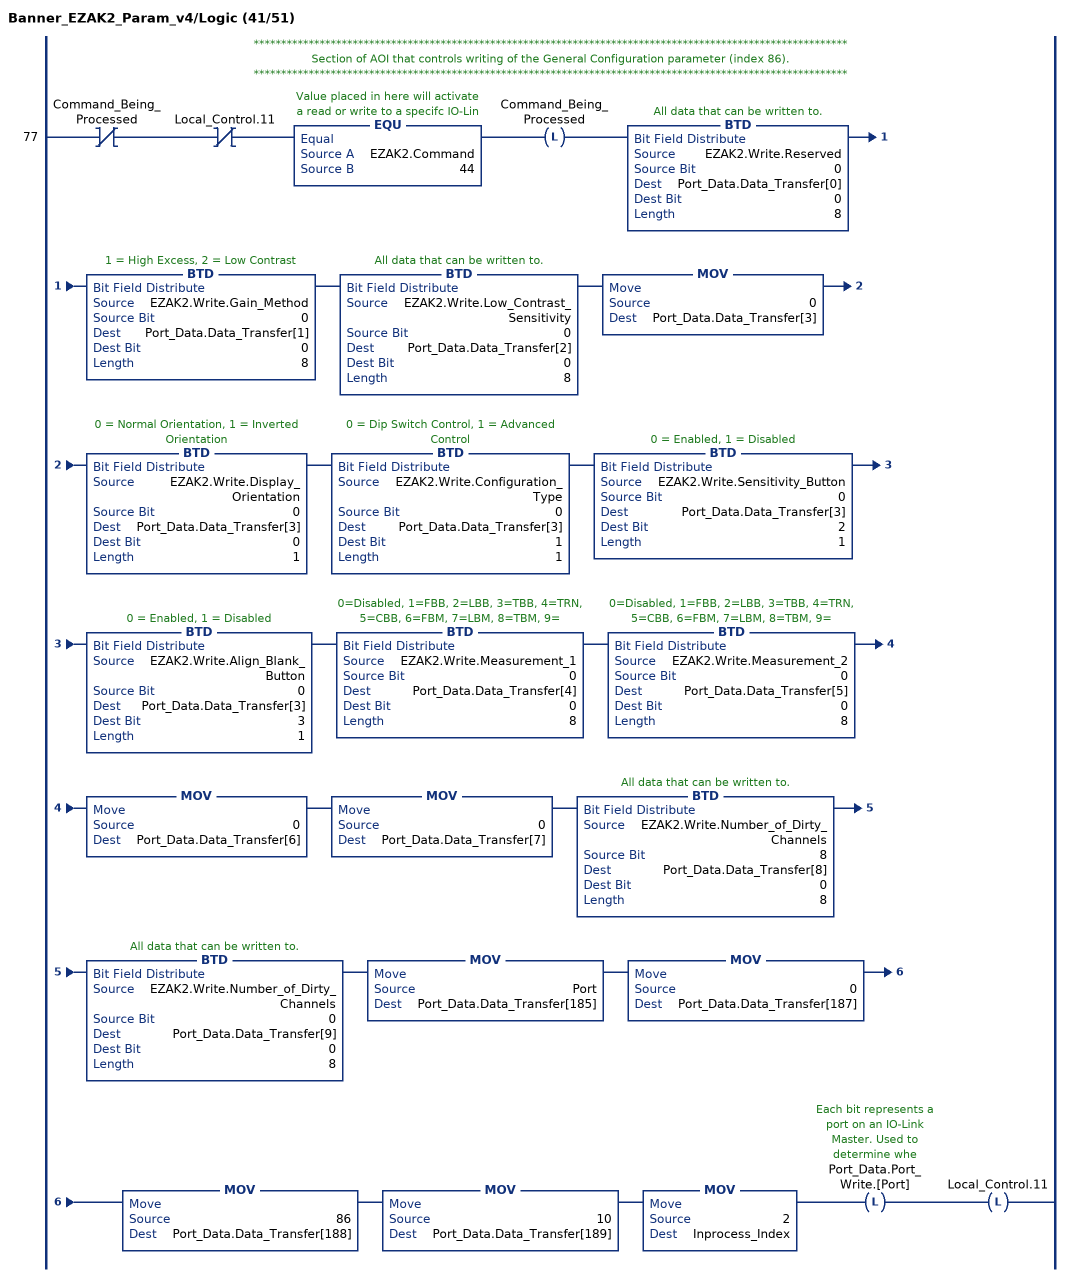
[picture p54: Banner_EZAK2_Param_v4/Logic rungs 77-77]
   // ************************************************************************************************************
   // Section of AOI that controls writing of the General Configuration parameter (index 86).
   // ************************************************************************************************************
   77: XIO(Command_Being_Processed)XIO(Local_Control.11)EQU(EZAK2.Command,44)OTL(Command_Being_Processed)BTD(EZAK2.Write.Reserved,0,Port_Data.Data_Transfer[0],0,8)BTD(EZAK2.Write.Gain_Method,0,Port_Data.Data_Transfer[1],0,8)BTD(EZAK2.Write.Low_Contrast_Sensitivity,0,Port_Data.Data_Transfer[2],0,8)MOV(0,Port_Data.Data_Transfer[3])BTD(EZAK2.Write.Display_Orientation,0,Port_Data.Data_Transfer[3],0,1)BTD(EZAK2.Write.Configuration_Type,0,Port_Data.Data_Transfer[3],1,1)BTD(EZAK2.Write.Sensitivity_Button,0,Port_Data.Data_Transfer[3],2,1)BTD(EZAK2.Write.Align_Blank_Button,0,Port_Data.Data_Transfer[3],3,1)BTD(EZAK2.Write.Measurement_1,0,Port_Data.Data_Transfer[4],0,8)BTD(EZAK2.Write.Measurement_2,0,Port_Data.Data_Transfer[5],0,8)MOV(0,Port_Data.Data_Transfer[6])MOV(0,Port_Data.Data_Transfer[7])BTD(EZAK2.Write.Number_of_Dirty_Channels,8,Port_Data.Data_Transfer[8],0,8)BTD(EZAK2.Write.Number_of_Dirty_Channels,0,Port_Data.Data_Transfer[9],0,8)MOV(Port,Port_Data.Data_Transfer[185])MOV(0,Port_Data.Data_Transfer[187])MOV(86,Port_Data.Data_Transfer[188])MOV(10,Port_Data.Data_Transfer[189])MOV(2,Inprocess_Index)OTL(Port_Data.Port_Write.[Port])OTL(Local_Control.11);
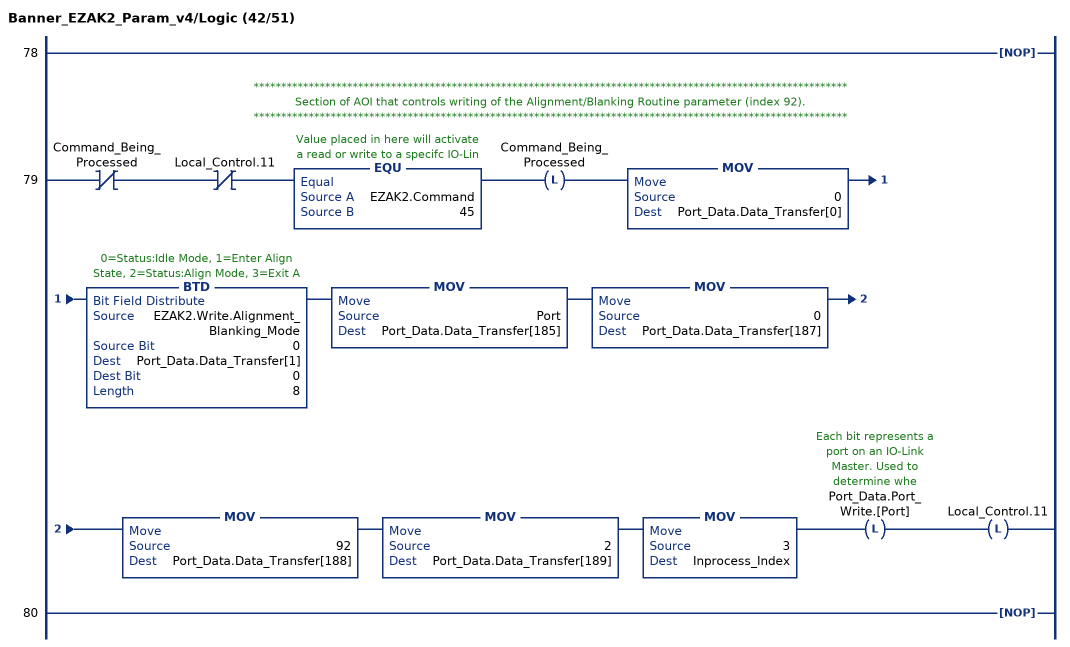
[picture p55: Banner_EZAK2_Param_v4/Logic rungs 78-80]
   78: NOP();
   // ************************************************************************************************************
   // Section of AOI that controls writing of the Alignment/Blanking Routine parameter (index 92).
   // ************************************************************************************************************
   79: XIO(Command_Being_Processed)XIO(Local_Control.11)EQU(EZAK2.Command,45)OTL(Command_Being_Processed)MOV(0,Port_Data.Data_Transfer[0])BTD(EZAK2.Write.Alignment_Blanking_Mode,0,Port_Data.Data_Transfer[1],0,8)MOV(Port,Port_Data.Data_Transfer[185])MOV(0,Port_Data.Data_Transfer[187])MOV(92,Port_Data.Data_Transfer[188])MOV(2,Port_Data.Data_Transfer[189])MOV(3,Inprocess_Index)OTL(Port_Data.Port_Write.[Port])OTL(Local_Control.11);
   80: NOP();
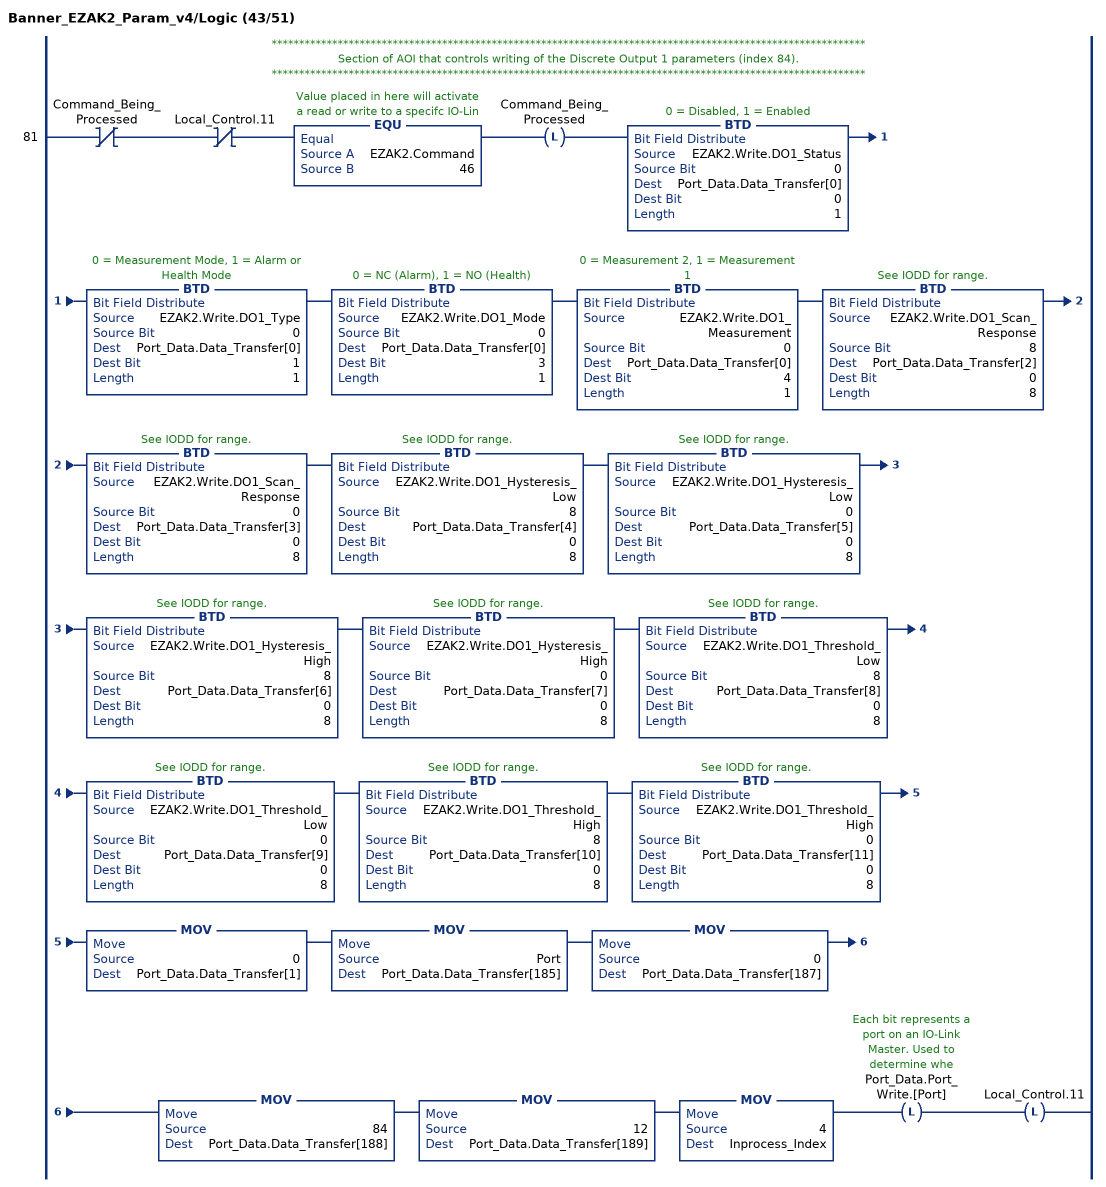
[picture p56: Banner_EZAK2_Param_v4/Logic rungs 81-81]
   // ************************************************************************************************************
   // Section of AOI that controls writing of the Discrete Output 1 parameters (index 84).
   // ************************************************************************************************************
   81: XIO(Command_Being_Processed)XIO(Local_Control.11)EQU(EZAK2.Command,46)OTL(Command_Being_Processed)BTD(EZAK2.Write.DO1_Status,0,Port_Data.Data_Transfer[0],0,1)BTD(EZAK2.Write.DO1_Type,0,Port_Data.Data_Transfer[0],1,1)BTD(EZAK2.Write.DO1_Mode,0,Port_Data.Data_Transfer[0],3,1)BTD(EZAK2.Write.DO1_Measurement,0,Port_Data.Data_Transfer[0],4,1)BTD(EZAK2.Write.DO1_Scan_Response,8,Port_Data.Data_Transfer[2],0,8)BTD(EZAK2.Write.DO1_Scan_Response,0,Port_Data.Data_Transfer[3],0,8)BTD(EZAK2.Write.DO1_Hysteresis_Low,8,Port_Data.Data_Transfer[4],0,8)BTD(EZAK2.Write.DO1_Hysteresis_Low,0,Port_Data.Data_Transfer[5],0,8)BTD(EZAK2.Write.DO1_Hysteresis_High,8,Port_Data.Data_Transfer[6],0,8)BTD(EZAK2.Write.DO1_Hysteresis_High,0,Port_Data.Data_Transfer[7],0,8)BTD(EZAK2.Write.DO1_Threshold_Low,8,Port_Data.Data_Transfer[8],0,8)BTD(EZAK2.Write.DO1_Threshold_Low,0,Port_Data.Data_Transfer[9],0,8)BTD(EZAK2.Write.DO1_Threshold_High,8,Port_Data.Data_Transfer[10],0,8)BTD(EZAK2.Write.DO1_Threshold_High,0,Port_Data.Data_Transfer[11],0,8)MOV(0,Port_Data.Data_Transfer[1])MOV(Port,Port_Data.Data_Transfer[185])MOV(0,Port_Data.Data_Transfer[187])MOV(84,Port_Data.Data_Transfer[188])MOV(12,Port_Data.Data_Transfer[189])MOV(4,Inprocess_Index)OTL(Port_Data.Port_Write.[Port])OTL(Local_Control.11);
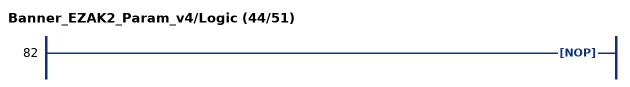
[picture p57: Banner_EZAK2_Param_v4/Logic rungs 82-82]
   82: NOP();
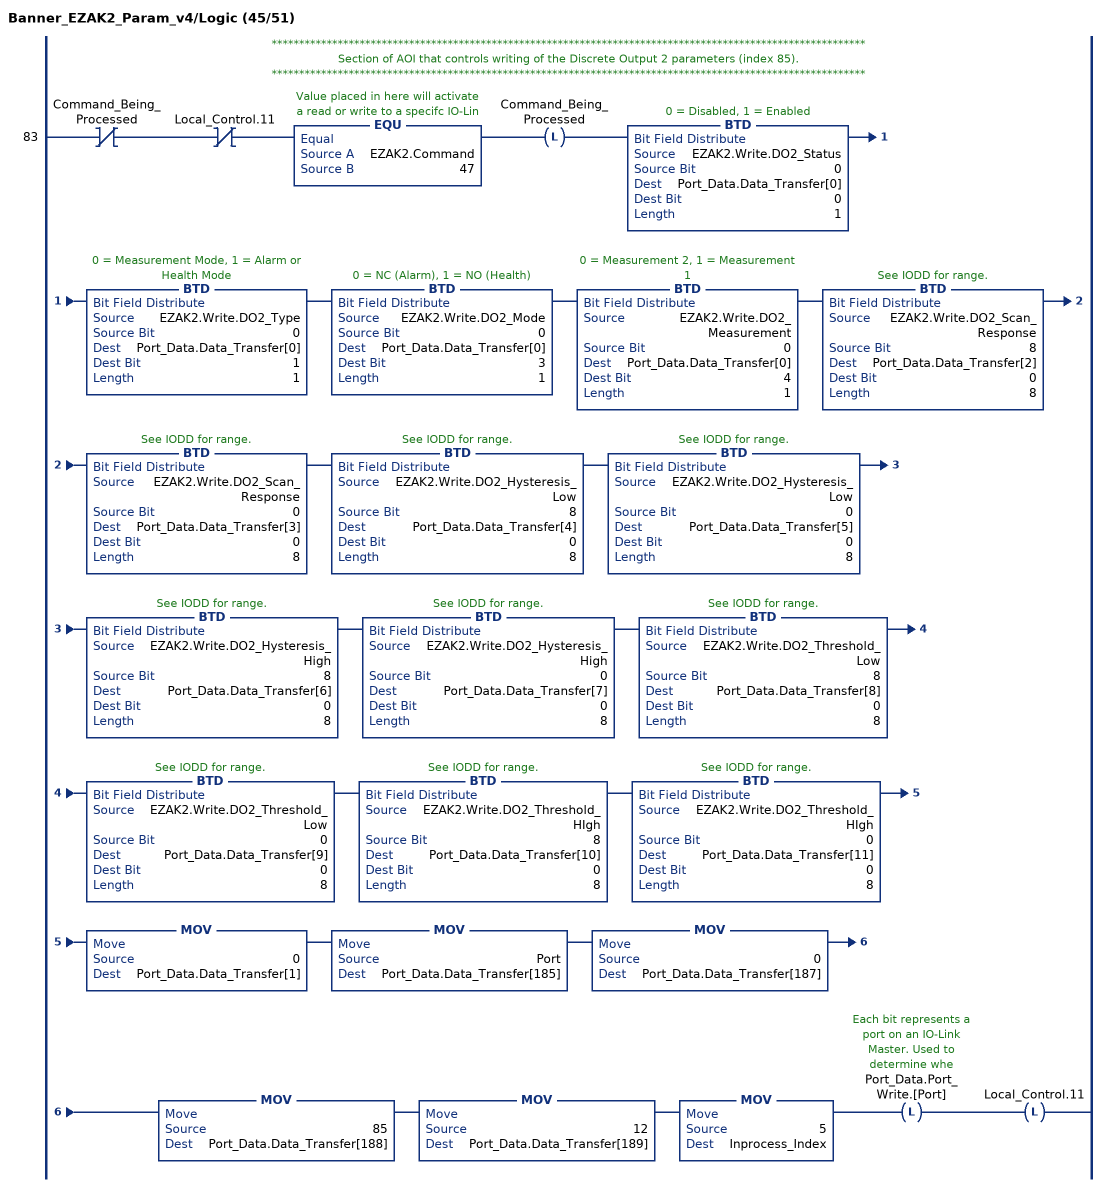
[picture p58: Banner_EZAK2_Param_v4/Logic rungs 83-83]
   // ************************************************************************************************************
   // Section of AOI that controls writing of the Discrete Output 2 parameters (index 85).
   // ************************************************************************************************************
   83: XIO(Command_Being_Processed)XIO(Local_Control.11)EQU(EZAK2.Command,47)OTL(Command_Being_Processed)BTD(EZAK2.Write.DO2_Status,0,Port_Data.Data_Transfer[0],0,1)BTD(EZAK2.Write.DO2_Type,0,Port_Data.Data_Transfer[0],1,1)BTD(EZAK2.Write.DO2_Mode,0,Port_Data.Data_Transfer[0],3,1)BTD(EZAK2.Write.DO2_Measurement,0,Port_Data.Data_Transfer[0],4,1)BTD(EZAK2.Write.DO2_Scan_Response,8,Port_Data.Data_Transfer[2],0,8)BTD(EZAK2.Write.DO2_Scan_Response,0,Port_Data.Data_Transfer[3],0,8)BTD(EZAK2.Write.DO2_Hysteresis_Low,8,Port_Data.Data_Transfer[4],0,8)BTD(EZAK2.Write.DO2_Hysteresis_Low,0,Port_Data.Data_Transfer[5],0,8)BTD(EZAK2.Write.DO2_Hysteresis_High,8,Port_Data.Data_Transfer[6],0,8)BTD(EZAK2.Write.DO2_Hysteresis_High,0,Port_Data.Data_Transfer[7],0,8)BTD(EZAK2.Write.DO2_Threshold_Low,8,Port_Data.Data_Transfer[8],0,8)BTD(EZAK2.Write.DO2_Threshold_Low,0,Port_Data.Data_Transfer[9],0,8)BTD(EZAK2.Write.DO2_Threshold_HIgh,8,Port_Data.Data_Transfer[10],0,8)BTD(EZAK2.Write.DO2_Threshold_HIgh,0,Port_Data.Data_Transfer[11],0,8)MOV(0,Port_Data.Data_Transfer[1])MOV(Port,Port_Data.Data_Transfer[185])MOV(0,Port_Data.Data_Transfer[187])MOV(85,Port_Data.Data_Transfer[188])MOV(12,Port_Data.Data_Transfer[189])MOV(5,Inprocess_Index)OTL(Port_Data.Port_Write.[Port])OTL(Local_Control.11);
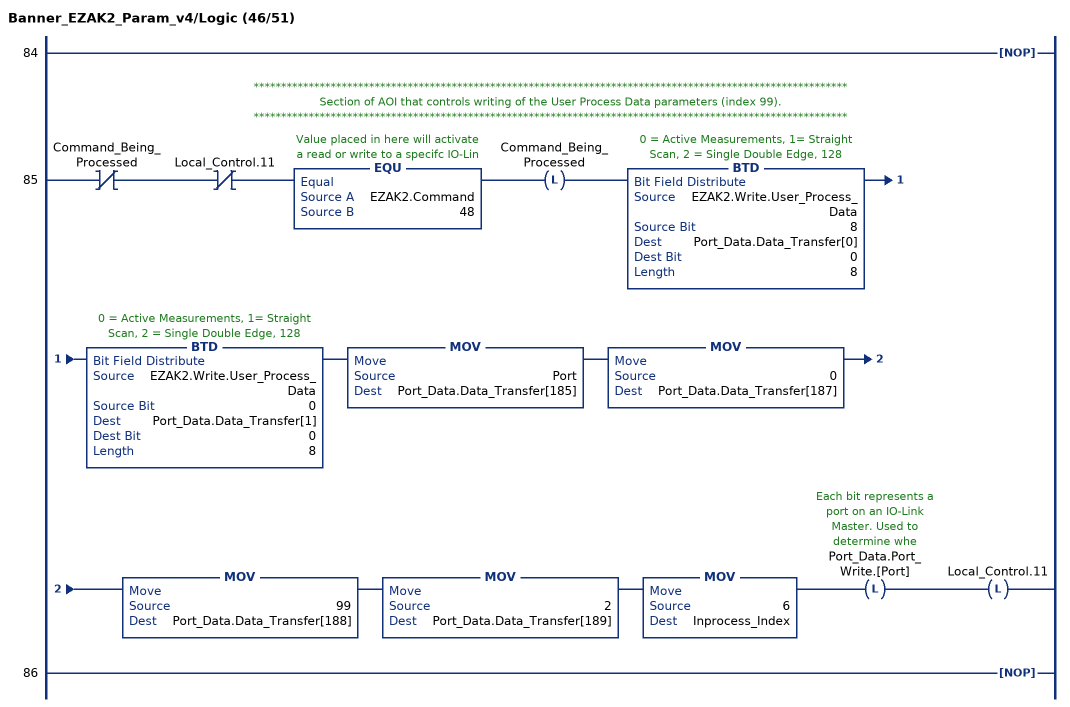
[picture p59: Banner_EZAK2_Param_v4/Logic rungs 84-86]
   84: NOP();
   // ************************************************************************************************************
   // Section of AOI that controls writing of the User Process Data parameters (index 99).
   // ************************************************************************************************************
   85: XIO(Command_Being_Processed)XIO(Local_Control.11)EQU(EZAK2.Command,48)OTL(Command_Being_Processed)BTD(EZAK2.Write.User_Process_Data,8,Port_Data.Data_Transfer[0],0,8)BTD(EZAK2.Write.User_Process_Data,0,Port_Data.Data_Transfer[1],0,8)MOV(Port,Port_Data.Data_Transfer[185])MOV(0,Port_Data.Data_Transfer[187])MOV(99,Port_Data.Data_Transfer[188])MOV(2,Port_Data.Data_Transfer[189])MOV(6,Inprocess_Index)OTL(Port_Data.Port_Write.[Port])OTL(Local_Control.11);
   86: NOP();
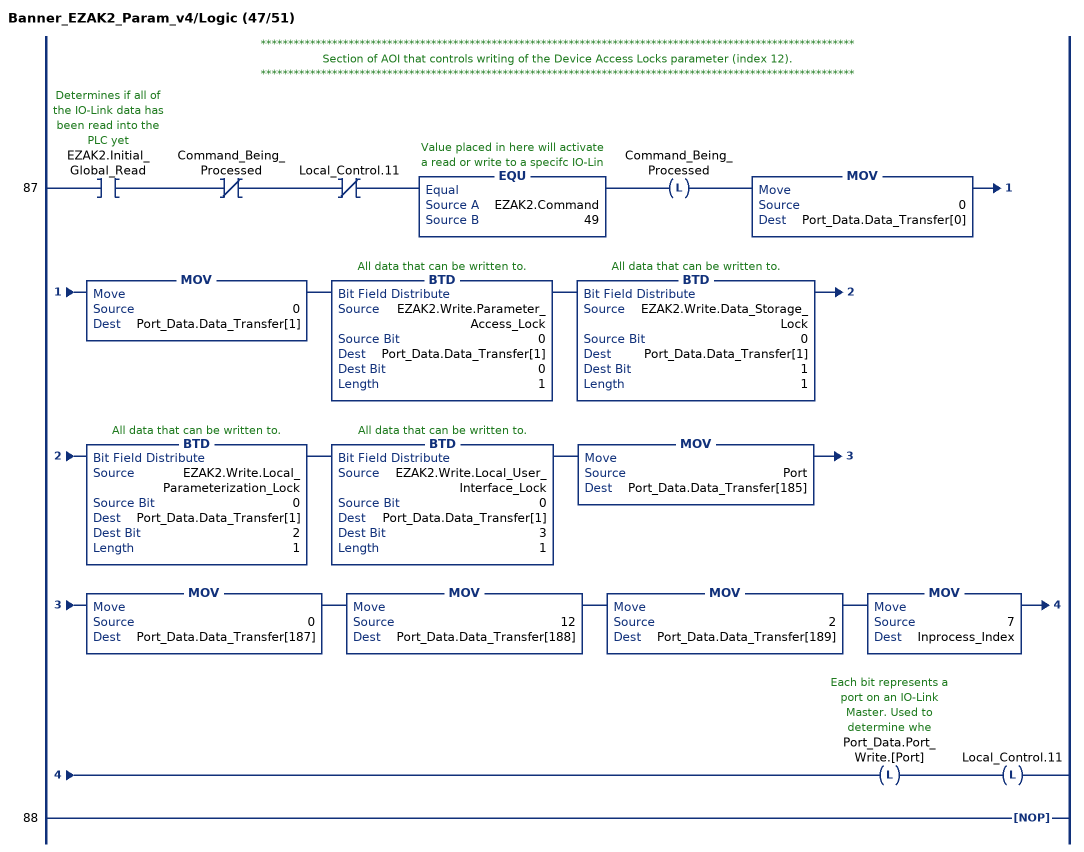
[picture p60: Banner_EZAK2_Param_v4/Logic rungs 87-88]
   // ************************************************************************************************************
   // Section of AOI that controls writing of the Device Access Locks parameter (index 12).
   // ************************************************************************************************************
   87: XIC(EZAK2.Initial_Global_Read)XIO(Command_Being_Processed)XIO(Local_Control.11)EQU(EZAK2.Command,49)OTL(Command_Being_Processed)MOV(0,Port_Data.Data_Transfer[0])MOV(0,Port_Data.Data_Transfer[1])BTD(EZAK2.Write.Parameter_Access_Lock,0,Port_Data.Data_Transfer[1],0,1)BTD(EZAK2.Write.Data_Storage_Lock,0,Port_Data.Data_Transfer[1],1,1)BTD(EZAK2.Write.Local_Parameterization_Lock,0,Port_Data.Data_Transfer[1],2,1)BTD(EZAK2.Write.Local_User_Interface_Lock,0,Port_Data.Data_Transfer[1],3,1)MOV(Port,Port_Data.Data_Transfer[185])MOV(0,Port_Data.Data_Transfer[187])MOV(12,Port_Data.Data_Transfer[188])MOV(2,Port_Data.Data_Transfer[189])MOV(7,Inprocess_Index)OTL(Port_Data.Port_Write.[Port])OTL(Local_Control.11);
   88: NOP();
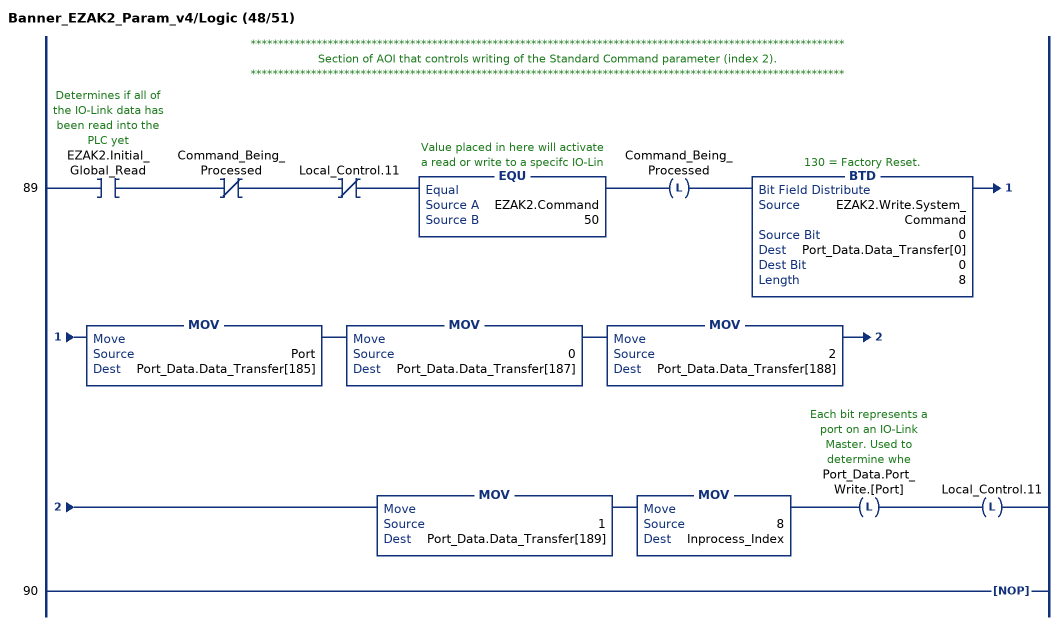
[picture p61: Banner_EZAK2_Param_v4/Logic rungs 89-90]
   // ************************************************************************************************************
   // Section of AOI that controls writing of the Standard Command parameter (index 2).
   // ************************************************************************************************************
   89: XIC(EZAK2.Initial_Global_Read)XIO(Command_Being_Processed)XIO(Local_Control.11)EQU(EZAK2.Command,50)OTL(Command_Being_Processed)BTD(EZAK2.Write.System_Command,0,Port_Data.Data_Transfer[0],0,8)MOV(Port,Port_Data.Data_Transfer[185])MOV(0,Port_Data.Data_Transfer[187])MOV(2,Port_Data.Data_Transfer[188])MOV(1,Port_Data.Data_Transfer[189])MOV(8,Inprocess_Index)OTL(Port_Data.Port_Write.[Port])OTL(Local_Control.11);
   90: NOP();
